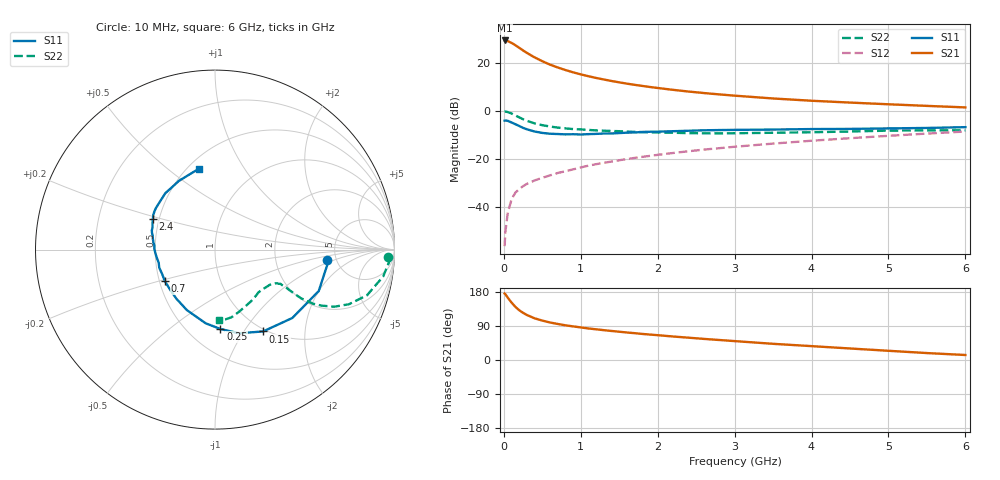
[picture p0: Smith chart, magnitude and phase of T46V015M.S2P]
! Infineon Technologies  Discrete & RF Semiconductors
! BFR182T
! Si NPN RF Bipolar Junction Transistor in SC75
! VCE = 6 V  IC = 15 mA
! Common Emitter S-Parameters:  October  1999
# GHz  S  MA  R  50
!  f  S11  S21  S12  S22
! GHz  MAG  ANG  MAG  ANG  MAG  ANG  MAG  ANG
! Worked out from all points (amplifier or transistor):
!   36 points, 10 MHz to 6 GHz, reference 50 ohm
!   highest |S21| = 29.4 dB at 10 MHz (marker M1)
!   |S21| within 3 dB of that: start of sweep to 197 MHz
!   unconditionally stable (mu >= 1): 846.5 MHz to 3.788 GHz
!   at 250 MHz: K = 0.54, MSG = 28.3 dB, |S12| = -31.4 dB
!   at 1.4 GHz: K = 1.08, MAG = 15.1 dB, |S12| = -21.1 dB
!   at 6 GHz: K = 0.86, MSG = 5.0 dB, |S12| = -8.6 dB
!   S11 on the Smith chart (normalised r, x): 10 MHz: 4.20, -0.82; 150 MHz: 0.97, -1.23; 250 MHz: 0.71, -0.78; 700 MHz: 0.53, -0.21; 2.4 GHz: 0.46, +0.19; 6 GHz: 0.57, +0.65
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0.01  0.6272 -5.4  29.67 175.4  0.0015 74.5  0.965 -2.5
0.02  0.632 -7.4  29.43 173.7  0.003 89.9  0.9748 -3.7
0.05  0.6224 -21.8  28.8 164.7  0.0072 80.9  0.9487 -9.1
0.1  0.5751 -41.5  26.42 151.6  0.0143 75.8  0.8846 -16.7
0.15  0.5289 -59.5  23.59 140.2  0.0197 68.2  0.8058 -22.2
0.2  0.4854 -73.9  20.85 131.4  0.0233 66.8  0.7364 -25.6
0.25  0.4432 -86.1  18.34 124.4  0.0269 62.1  0.6721 -27.7
0.3  0.414 -97.2  16.29 118.7  0.03 61.9  0.6238 -28.9
0.4  0.3718 -114.9  13.14 110.0  0.0354 61.6  0.5495 -29.5
0.5  0.348 -128.2  10.92 104.0  0.0402 62.6  0.5047 -29.0
0.6  0.3345 -139.3  9.289 99.0  0.0451 63.5  0.4731 -28.6
0.7  0.3298 -147.8  8.097 95.1  0.0506 65.1  0.4495 -28.1
0.9  0.3267 -162.0  6.407 88.7  0.0602 66.5  0.4185 -27.8
1.1  0.3282 -172.7  5.313 83.2  0.0721 67.5  0.4017 -28.3
1.3  0.3382 179.3  4.541 78.7  0.0828 68.1  0.3864 -29.2
1.6  0.3522 169.7  3.719 72.6  0.0989 68.3  0.3707 -31.2
2.2  0.3776 157.2  2.76 62.0  0.1325 68.0  0.3506 -37.5
2.4  0.3859 153.8  2.545 58.9  0.1439 67.8  0.3442 -40.0
3.5  0.4085 137.6  1.822 42.7  0.208 63.8  0.3504 -54.6
4.5  0.4217 125.1  1.496 30.4  0.2699 59.0  0.3722 -69.3
5.5  0.4415 109.2  1.276 18.3  0.3367 53.3  0.3931 -81.7
6  0.4589 101.5  1.186 13.2  0.3717 49.8  0.3938 -86.6
